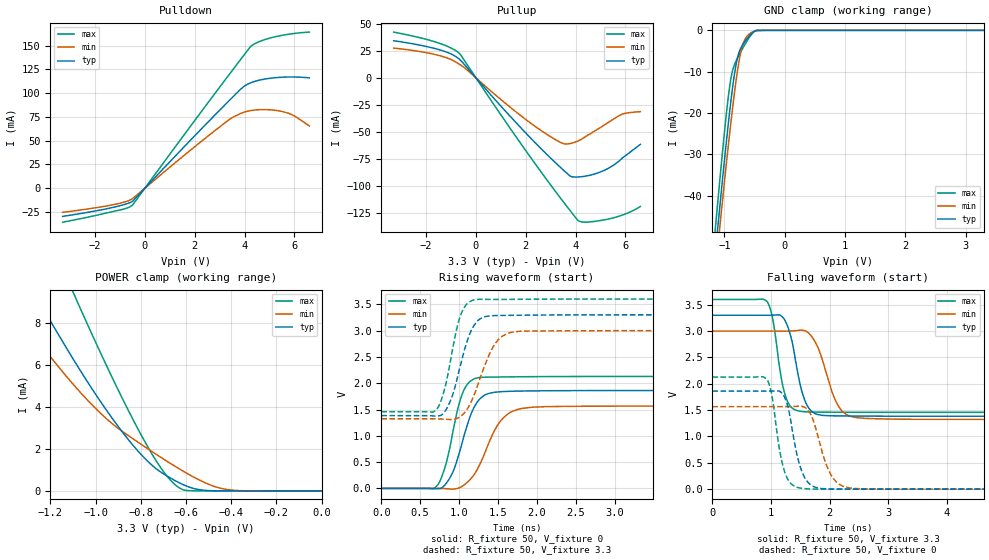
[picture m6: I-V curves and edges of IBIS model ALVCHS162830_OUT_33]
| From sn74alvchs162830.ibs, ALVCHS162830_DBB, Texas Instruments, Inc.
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[Model]   ALVCHS162830_OUT_33
Model_type  3-state
Enable   Active-Low
Vref =   0.0
Rref =   500
Cref =   50p
Vmeas =   1.5
| variable   typ   min   max
C_comp   3.82pF   2.46pF   6.12pF
| C_pullup   3.29pF   2.56pF   4.78pF
| C_pulldown   2.92pF   2.46pF   3.78pF
| C_tri-state   5.25pF   4.42pF   6.12pF
[Temperature Range]   40   100   -40
| Ambient temperature   25   85   -40
[Voltage range]   3.3   3   3.6
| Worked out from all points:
|   slope of the pulldown table from 0 to 0.495 V, typ, clamps not added: 35.9 ohm
|   slope of the pullup table from 0 to 0.495 V, typ, clamps not added: 37.9 ohm
|   GND clamp passes 1 mA (typ) near -0.56 V on its own axis
|   POWER clamp passes 1 mA (typ) near -0.72 V on its own axis
|   rising waveform, R_fixture 50, V_fixture 0: 20-80 % time 239ps typ, 304ps min, 196ps max; typ from 0 V to 1.86 V
|   falling waveform, R_fixture 50, V_fixture 3.3: 20-80 % time 219ps typ, 301ps min, 179ps max; typ from 3.3 V to 1.38 V
|   rising waveform, R_fixture 50, V_fixture 3.3: 20-80 % time 217ps typ, 269ps min, 181ps max; typ from 1.38 V to 3.3 V
|   falling waveform, R_fixture 50, V_fixture 0: 20-80 % time 210ps typ, 266ps min, 180ps max; typ from 1.86 V to 0 V
[GND Clamp]
| ALVCHS162830_OUT_33
|   Voltage   I(typ)   I(min)   I(max)
-3.3V     -404.3mA   -397.8mA   -415.1mA
-1.16V    -55.3mA    -59.85mA   -49.53mA
-1.14V    -52.25mA   -56.9mA    -46.31mA
-1.1V     -46.21mA   -51.04mA   -39.95mA
-1.08V    -43.22mA   -48.14mA   -36.81mA
-1.065V   -40.99mA   -45.98mA   -34.48mA
-915mV    -19.95mA   -25.2mA    -13.81mA
-865mV    -13.89mA   -18.85mA   -9.751mA
-800mV    -7.763mA   -11.44mA   -7.198mA
-685mV    -3.203mA   -3.029mA   -4.054mA
-495mV    -129.9uA   -257.4uA   -143.7uA
3.3V      79.44pA    2.143uA    7.942pA
[POWER Clamp]
| ALVCHS162830_OUT_33
|   Voltage   I(typ)   I(min)   I(max)
-3.3V     55.35mA    43.9mA     72.91mA
-1.41V    12.15mA    9.436mA    17.4mA
-1.265V   9.314mA    7.293mA    13.61mA
-1.11V    6.47mA     5.212mA    9.72mA
-1.085V   6.033mA    4.903mA    9.111mA
-960mV    3.97mA     3.517mA    6.158mA
-830mV    2.118mA    2.449mA    3.309mA
-730mV    1.041mA    1.729mA    1.402mA
-645mV    470.9uA    1.15mA     268.5uA
-600mV    241.3uA    862.7uA    23.2uA
-430mV    1.282uA    87.65uA    28.07nA
-48.03fV  79.44pA    405.7pA    9.202pA
[Pulldown]
| ALVCHS162830_OUT_33
|   Voltage   I(typ)   I(min)   I(max)
-3.3V     -29.65mA   -25.37mA   -35.72mA
-1.365V   -20.67mA   -17.82mA   -25.01mA
-790mV    -16.89mA   -14.29mA   -21.48mA
-525mV    -14.22mA   -11.37mA   -18.3mA
1.78V     49.15mA    38.97mA    63.42mA
3.36V     91.58mA    71.69mA    118.8mA
3.895V    105.4mA    79.21mA    137.3mA
4.245V    110.9mA    81.7mA     149mA
4.755V    114.6mA    82.74mA    155.8mA
5.6V      116.9mA    80.13mA    161.3mA
5.995V    117mA      76.15mA    162.8mA
6.6V      116.1mA    65.53mA    164.3mA
[Pullup]
| ALVCHS162830_OUT_33
|   Voltage   I(typ)   I(min)   I(max)
-3.3V     34.27mA    27.49mA    42.27mA
-1.495V   26.13mA    20.74mA    32.17mA
-985mV    21.93mA    16.8mA     27.39mA
-665mV    17.14mA    12.56mA    22.56mA
2.405V    -60.63mA   -45.35mA   -80.33mA
3.41V     -83.18mA   -59.89mA   -111.7mA
3.81V     -91.16mA   -60.62mA   -123.6mA
4.12V     -91.67mA   -58.12mA   -132.2mA
4.505V    -90.43mA   -52.88mA   -133.4mA
5.235V    -84.62mA   -42.44mA   -131mA
5.825V    -75.23mA   -34.01mA   -127.3mA
6.6V      -61.55mA   -31.31mA   -119mA
[Ramp]
| ALVCHS162830_OUT_33
| variable   typ   min   max
dV/dt_r   1.12/2.48E-10   0.95/3.18E-10   1.28/1.97E-10
dV/dt_f   1.16/2.24E-10   1.02/3.14E-10   1.29/1.84E-10
R_load = 50
[Rising Waveform]
| ALVCHS162830_OUT_33
R_fixture =   50
C_fixture =   0
L_fixture =   0
V_fixture =   0
V_fixture_min = 0
V_fixture_max = 0
|   Time   V(typ)   V(min)   V(max)
0s        -2.006uV   -7.418uV   -385.2nV
715ps     -5.752mV   903.6uV    48.73mV
815ps     60.08mV    -3.936mV   383.2mV
900ps     249.6mV    -14.08mV   917.2mV
1.055ns   951.7mV    55.99mV    1.847V
1.19ns    1.532V     255.5mV    2.08V
1.34ns    1.782V     705.6mV    2.115V
1.655ns   1.846V     1.442V     2.121V
2.35ns    1.859V     1.559V     2.127V
50ns      1.86V      1.565V     2.128V
[Falling Waveform]
| ALVCHS162830_OUT_33
R_fixture =   50
C_fixture =   0
L_fixture =   0
V_fixture =   3.3
V_fixture_min = 3
V_fixture_max = 3.6
|   Time   V(typ)   V(min)   V(max)
0s        3.3V       3V         3.6V
935ps     3.3V       3V         3.56V
1.035ns   3.302V     3V         3.197V
1.195ns   3.268V     2.999V     1.997V
1.34ns    2.889V     3.001V     1.561V
1.51ns    1.929V     3.018V     1.476V
1.65ns    1.531V     2.954V     1.464V
2.195ns   1.389V     1.506V     1.459V
2.82ns    1.385V     1.335V     1.458V
50ns      1.384V     1.324V     1.458V
[Rising Waveform]
| ALVCHS162830_OUT_33
R_fixture =   50
C_fixture =   0
L_fixture =   0
V_fixture =   3.3
V_fixture_min = 3
V_fixture_max = 3.6
|   Time   V(typ)   V(min)   V(max)
0s        1.384V     1.324V     1.458V
710ps     1.377V     1.322V     1.504V
790ps     1.416V     1.318V     1.768V
870ps     1.602V     1.312V     2.274V
1.025ns   2.382V     1.375V     3.314V
1.14ns    2.948V     1.601V     3.551V
1.26ns    3.213V     2.05V      3.596V
1.52ns    3.288V     2.851V     3.593V
1.935ns   3.295V     2.994V     3.598V
50ns      3.3V       3V         3.6V
[Falling Waveform]
| ALVCHS162830_OUT_33
R_fixture =   50
C_fixture =   0
L_fixture =   0
V_fixture =   0
V_fixture_min = 0
V_fixture_max = 0
|   Time   V(typ)   V(min)   V(max)
0s        1.86V      1.565V     2.128V
935ps     1.861V     1.565V     2.079V
1.015ns   1.861V     1.565V     1.784V
1.175ns   1.834V     1.565V     578.5mV
1.335ns   1.315V     1.567V     111mV
1.49ns    456.6mV    1.577V     23.05mV
1.665ns   92.44mV    1.443V     3.342mV
2.045ns   2.285mV    233.5mV    576.9uV
2.525ns   875.9uV    7.007mV    251.1uV
50ns      -2.002uV   -7.314uV   -377nV
